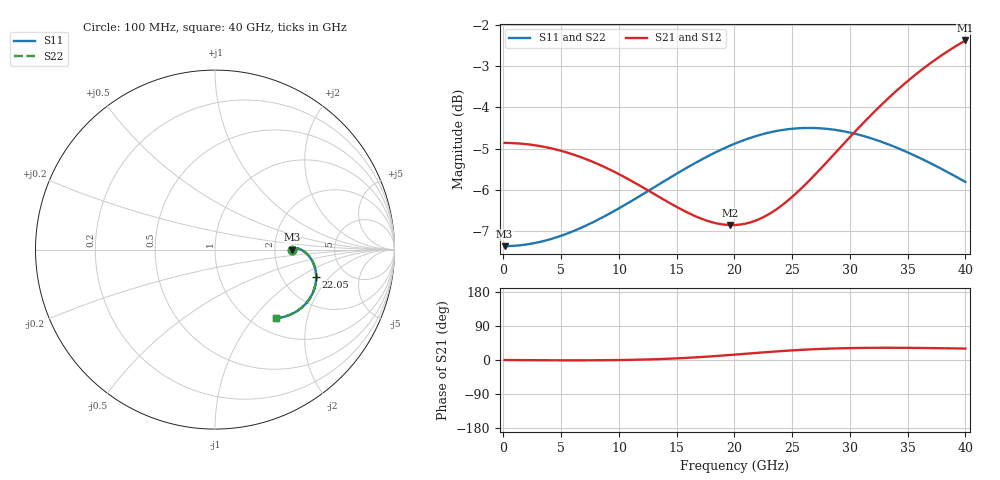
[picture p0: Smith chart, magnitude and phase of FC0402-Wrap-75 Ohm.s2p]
!Vishay Thin-Film
!FC Family
!Case Size 0402
!Assembly Style Full Wrap SMT
!10/21/2015
!thinfilm@vishay.com
# GHz S MA R 50
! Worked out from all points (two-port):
!   101 points, 100 MHz to 40 GHz, reference 50 ohm
!   highest |S21| = -2.38 dB at 40 GHz (marker M1); lowest = -6.8 dB at 19.65 GHz (marker M2)
!   |S21| within 3 dB of the highest: start of sweep to 8.253 GHz; 27.81 GHz to end of sweep
!   lowest |S11| = -7.4 dB at 100 MHz (marker M3), VSWR 2.50, Z = 125 + j0.0628 ohm
!   |S11| at or under -10 dB: nowhere
!   |S22| runs from -7.4 to -4.5 dB; largest |S21 - S12| = 0
!   S11 on the Smith chart (normalised r, x): 100 MHz: 2.50, +0.00; 22.05 GHz: 3.10, -1.41; 40 GHz: 1.28, -1.32
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0.1  0.4286 0.0  0.5714 -0.0  0.5714 -0.0  0.4286 0.0
3.292  0.4341 0.8  0.566 -0.6  0.566 -0.6  0.4341 0.8
6.883  0.4521 1.0  0.548 -0.8  0.548 -0.8  0.4521 1.0
8.878  0.4668 0.6  0.5333 -0.5  0.5333 -0.5  0.4668 0.6
10.474  0.4804 -0.1  0.5196 0.1  0.5196 0.1  0.4804 -0.1
12.07  0.4954 -1.1  0.5048 1.1  0.5048 1.1  0.4954 -1.1
13.666  0.5111 -2.5  0.4899 2.6  0.4899 2.6  0.5111 -2.5
16.459  0.5389 -5.7  0.4669 6.6  0.4669 6.6  0.5389 -5.7
18.055  0.5538 -8.0  0.4582 9.7  0.4582 9.7  0.5538 -8.0
19.651  0.5673 -10.6  0.4545 13.3  0.4545 13.3  0.5673 -10.6
20.05  0.5704 -11.3  0.4546 14.2  0.4546 14.2  0.5704 -11.3
22.045  0.5834 -14.9  0.4614 19.0  0.4614 19.0  0.5834 -14.9
23.242  0.5892 -17.2  0.4709 21.8  0.4709 21.8  0.5892 -17.2
24.439  0.5932 -19.6  0.4842 24.3  0.4842 24.3  0.5932 -19.6
26.833  0.5957 -24.5  0.5205 28.4  0.5205 28.4  0.5957 -24.5
28.429  0.5933 -27.8  0.5498 30.2  0.5498 30.2  0.5933 -27.8
30.424  0.5863 -31.8  0.5892 31.6  0.5892 31.6  0.5863 -31.8
32.02  0.5777 -34.9  0.6214 32.1  0.6214 32.1  0.5777 -34.9
33.616  0.5671 -37.9  0.6528 32.2  0.6528 32.2  0.5671 -37.9
35.212  0.5549 -40.7  0.6827 32.0  0.6827 32.0  0.5549 -40.7
36.808  0.5414 -43.3  0.7107 31.5  0.7107 31.5  0.5414 -43.3
40  0.5126 -48.1  0.7602 30.1  0.7602 30.1  0.5126 -48.1
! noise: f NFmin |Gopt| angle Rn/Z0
0.1  4.822e-15  1  -2.695e-17  1.5
4.489  1.43e-07  1  -2.372e-15  1.563
8.878  -3.857e-15  1  -4.992e-17  1.75
13.27  -2.411e-15  1  4.181e-15  2.049
17.66  6.75e-15  1  3.274e-15  2.296
22.05  0  1  -1.424e-14  2.098
26.43  1.322e-07  1  6.259e-15  1.444
30.82  7.742e-08  1  2.635e-15  0.846
35.21  -4.822e-16  1  -8.538e-07  0.4849
40  0  1  -2.495e-15  0.2757
